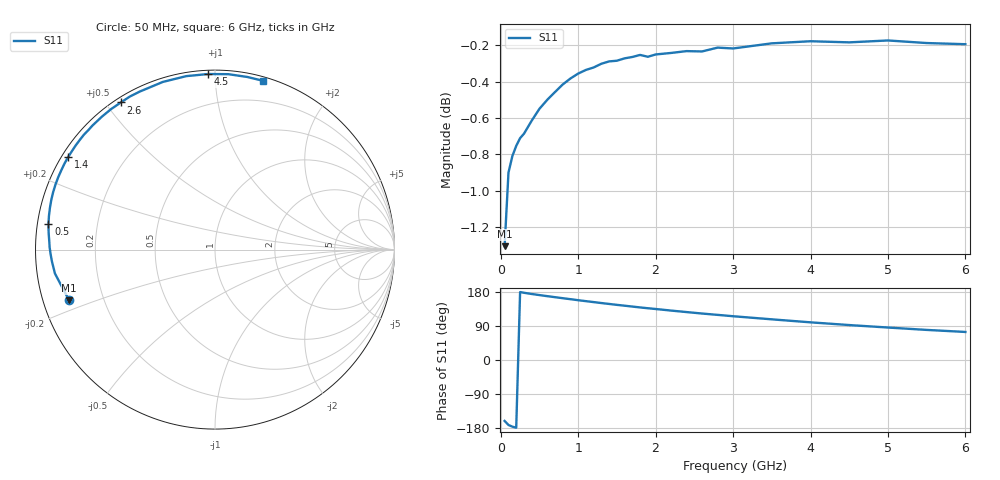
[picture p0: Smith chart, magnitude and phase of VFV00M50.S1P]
! Infineon Technologies  Discrete & RF Semiconductors
! BBY 58-03
! Si Tuning Diode in SOD323
! VR =
! S-Parameters:  June  1999
# GHz  S  MA  R  50
!  f  S11
! GHz  MAG  ANG
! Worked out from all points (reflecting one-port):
!   34 points, 50 MHz to 6 GHz, reference 50 ohm
!   lowest |S11| = -1.3 dB at 50 MHz (marker M1), VSWR 13.35, Z = 3.85 - j8.41 ohm
!   phase of S11 starts at -161 deg and turns -125 deg over the sweep
!   S11 on the Smith chart (normalised r, x): 50 MHz: 0.08, -0.17; 500 MHz: 0.03, +0.08; 1.4 GHz: 0.02, +0.29; 2.6 GHz: 0.02, +0.55; 4.5 GHz: 0.02, +0.96; 6 GHz: 0.03, +1.33
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0.05  0.8606 -160.8
0.1  0.9016 -171.5
0.15  0.911 -175.9
0.2  0.917 -178.7
0.25  0.9214 179.2
0.4  0.9317 174.2
0.5  0.9387 171.3
0.6  0.944 168.5
0.8  0.9532 163.1
0.9  0.9568 160.5
1  0.9598 157.8
1.1  0.962 155.3
1.4  0.9673 147.9
1.6  0.9691 143.3
1.8  0.9712 138.7
1.9  0.9701 136.6
2  0.9715 134.6
2.2  0.9724 130.4
2.4  0.9736 126.5
2.6  0.9734 122.6
2.8  0.9757 119.1
3  0.9752 115.5
3.5  0.9784 107.3
4  0.9797 99.4
4.5  0.979 92.2
5  0.9801 85.7
5.5  0.9785 79.4
6  0.9778 74.0
